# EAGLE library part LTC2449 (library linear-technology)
24-Bit High Speed 8-/16-Channel ΔΣ ADCs with Selectable Speed/Resolution Source: Data sheet
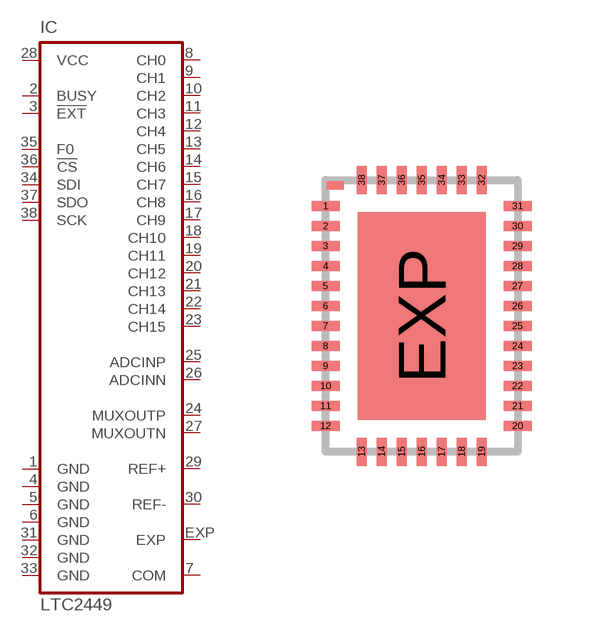
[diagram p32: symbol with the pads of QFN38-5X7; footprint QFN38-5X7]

Designator prefix IC

## LTC2449CUHF, LTC2449IUHF  [QFN38-5X7]
1  GND  pwr
2  BUSY  out
3  !EXT  out
4  GND  pwr
5  GND  pwr
6  GND  pwr
7  COM  pwr
8  CH0  in
9  CH1  in
10  CH2  in
11  CH3  in
12  CH4  in
13  CH5  in
14  CH6  in
15  CH7  in
16  CH8  in
17  CH9  in
18  CH10  in
19  CH11  in
20  CH12  in
21  CH13  in
22  CH14  in
23  CH15  in
24  MUXOUTP  out
25  ADCINP  in
26  ADCINN  in
27  MUXOUTN  out
28  VCC  pwr
29  REF+  in
30  REF-  in
31  GND  pwr
32  GND  pwr
33  GND  pwr
34  SDI  in
35  F0  in
36  !CS  in
37  SDO  hiz
38  SCK
EXP  EXP  pas

## Footprint QFN38-5X7 (pad centres in mm)
UHF Package 38-Lead Plastic QFN (5mm × 7mm) (Reference LTC DWG # 05-08-1701) Source: Data sheet
smd 0.7 x 0.25: 1 -2.4,2.75; 2 -2.4,2.25; 3 -2.4,1.75; 4 -2.4,1.25; 5 -2.4,0.75; 6 -2.4,0.25; 7 -2.4,-0.25; 8 -2.4,-0.75; 9 -2.4,-1.25; 10 -2.4,-1.75; 11 -2.4,-2.25; 12 -2.4,-2.75; 20 2.4,-2.75; 21 2.4,-2.25; 22 2.4,-1.75; 23 2.4,-1.25; 24 2.4,-0.75; 25 2.4,-0.25; 26 2.4,0.25; 27 2.4,0.75; 28 2.4,1.25; 29 2.4,1.75; 30 2.4,2.25; 31 2.4,2.75
smd 0.25 x 0.7: 13 -1.5,-3.4; 14 -1,-3.4; 15 -0.5,-3.4; 16 0,-3.4; 17 0.5,-3.4; 18 1,-3.4; 19 1.5,-3.4; 32 1.5,3.4; 33 1,3.4; 34 0.5,3.4; 35 0,3.4; 36 -0.5,3.4; 37 -1,3.4; 38 -1.5,3.4
smd 3.2 x 5.2: EXP 0,0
